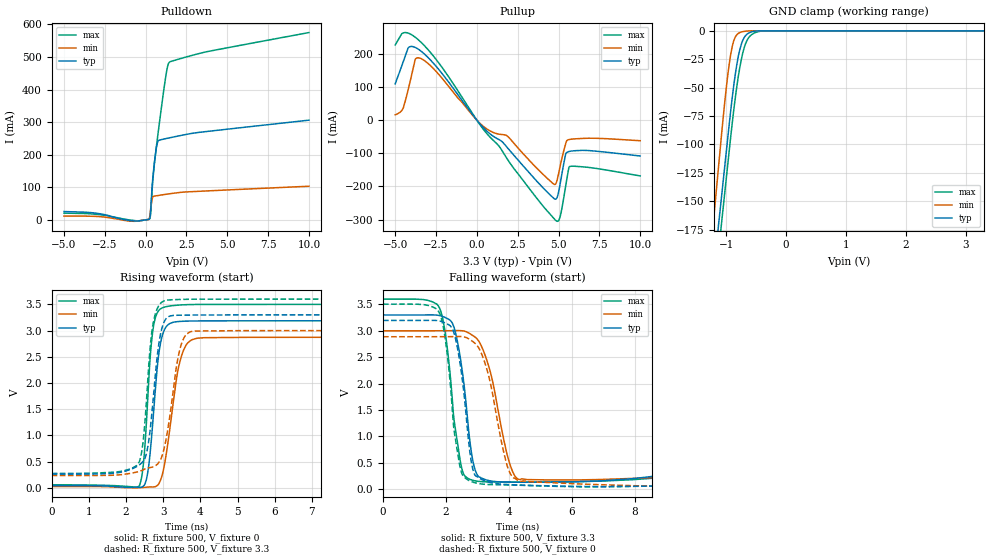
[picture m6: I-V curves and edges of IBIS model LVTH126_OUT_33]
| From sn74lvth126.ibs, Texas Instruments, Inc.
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[Model]   LVTH126_OUT_33
Model_type  3-state
Enable   Active-High
Vref =   0
Rref =   500
Cref =   50p
Vmeas =   1.5
| variable   typ   min   max
C_comp   3.41pF   2.80pF   4.69pF
| C_pullup   4.02pF   0.55pF   5.35pF
| C_pulldown   8.51pF   2.05pF   35.10pF
| C_tri-state   3.41pF   2.80pF   4.69pF
[Temperature Range]   40   -40   100
| Ambient temperature   25   -40   85
[Voltage range]   3.3   3   3.6
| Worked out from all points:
|   slope of the pulldown table from 0 to 0.495 V, typ, clamps not added: 3.18 ohm
|   slope of the pullup table from 0 to 0.495 V, typ, clamps not added: 17.9 ohm
|   GND clamp passes 1 mA (typ) near -0.58 V on its own axis
|   rising waveform, R_fixture 500, V_fixture 0: 20-80 % time 233ps typ, 344ps min, 188ps max; typ from 0.041 V to 3.19 V
|   falling waveform, R_fixture 500, V_fixture 3.3: 20-80 % time 371ps typ, 596ps min, 368ps max; typ from 3.3 V to 0.26 V
|   rising waveform, R_fixture 500, V_fixture 3.3: 20-80 % time 267ps typ, 353ps min, 220ps max; typ from 0.261 V to 3.3 V
|   falling waveform, R_fixture 500, V_fixture 0: 20-80 % time 369ps typ, 599ps min, 369ps max; typ from 3.2 V to 0.041 V
[GND Clamp]
| LVTH126_OUT_33
|   Voltage   I(typ)   I(min)   I(max)
-5.5V     -2.861A    -3.034A    -2.892A
-1.24V    -226.4mA   -182.9mA   -251mA
-1.21V    -211.3mA   -165.7mA   -235.5mA
-1.17V    -191.4mA   -142.9mA   -215.1mA
-1.075V   -144mA     -89.19mA   -167.4mA
-975mV    -94.37mA   -39.09mA   -117.7mA
-925mV    -69.94mA   -20.46mA   -92.96mA
-875mV    -48.14mA   -8.719mA   -69.85mA
-800mV    -22.75mA   -2.299mA   -40.47mA
-725mV    -8.466mA   -746.4uA   -19.69mA
-575mV    -873.9uA   -11.47uA   -3.26mA
3.3V      32.83pA    25.31pA    1.688nA
[Pulldown]
| LVTH126_OUT_33
|   Voltage   I(typ)   I(min)   I(max)
-5V       25.27mA    11.42mA    20.38mA
-3.085V   20.58mA    10.43mA    17.13mA
-705mV    -3.69mA    -4.657mA   -2.29mA
250mV     4.096mA    9.458mA    3.679mA
315mV     33.12mA    35.96mA    22.65mA
425mV     118.9mA    68.08mA    110mA
580mV     192.7mA    73.08mA    190.3mA
710mV     233.6mA    74.13mA    244.7mA
1.24V     249.3mA    78.23mA    442mA
1.36V     250.6mA    79.11mA    473.7mA
1.465V    251.7mA    79.87mA    484.4mA
10V       306mA      103.1mA    575.1mA
[Pullup]
| LVTH126_OUT_33
|   Voltage   I(typ)   I(min)   I(max)
-5V       110.1mA    16.64mA    227.5mA
-4.535V   173.3mA    34.41mA    263.2mA
-4.2V     218.9mA    93.95mA    263.1mA
-3.775V   219.9mA    183.8mA    250.7mA
-3.445V   209.6mA    186.9mA    236.7mA
260mV     -15.41mA   -12.72mA   -18.54mA
1.855V    -82.19mA   -47.41mA   -116.7mA
4.885V    -235.7mA   -185.5mA   -304.7mA
5.11V     -188.9mA   -136.1mA   -288.5mA
5.435V    -102.2mA   -70.96mA   -199.1mA
5.68V     -93.91mA   -57.89mA   -139.8mA
10V       -107.9mA   -61.81mA   -168.2mA
[Ramp]
| LVTH126_OUT_33
| variable   typ   min   max
dV/dt_r   1.91/2.38E-10   1.72/3.55E-10   2.10/1.92E-10
dV/dt_f   1.90/3.89E-10   1.70/6.11E-10   2.08/3.91E-10
R_load = 500
[Rising Waveform]
| LVTH126_OUT_33
R_fixture =   500
C_fixture =   0
L_fixture =   0
V_fixture =   0
V_fixture_min = 0
V_fixture_max = 0
|   Time   V(typ)   V(min)   V(max)
0s        41.24mV    24.56mV    57mV
2.36ns    10.18mV    941.8uV    40.3mV
2.465ns   31.77mV    5.651mV    442.3mV
2.57ns    234.3mV    12.17mV    1.515V
2.755ns   1.564V     17.13mV    3.143V
2.955ns   2.848V     200.1mV    3.426V
3.305ns   3.164V     1.809V     3.48V
3.595ns   3.179V     2.696V     3.493V
4.105ns   3.185V     2.864V     3.499V
50ns      3.188V     2.873V     3.5V
[Falling Waveform]
| LVTH126_OUT_33
R_fixture =   500
C_fixture =   0
L_fixture =   0
V_fixture =   3.3
V_fixture_min = 3
V_fixture_max = 3.6
|   Time   V(typ)   V(min)   V(max)
0s        3.3V       3V         3.6V
1.75ns    3.294V     3.001V     3.478V
1.98ns    3.251V     3.001V     2.95V
2.205ns   3.144V     3.002V     1.676V
2.53ns    2.187V     2.999V     334.1mV
2.81ns    690.5mV    2.927V     175.3mV
3.025ns   245.2mV    2.819V     148.1mV
3.995ns   133.2mV    542.3mV    135.5mV
4.33ns    130.9mV    183.6mV    135.1mV
50ns      260.2mV    234.4mV    273.1mV
[Rising Waveform]
| LVTH126_OUT_33
R_fixture =   500
C_fixture =   0
L_fixture =   0
V_fixture =   3.3
V_fixture_min = 3
V_fixture_max = 3.6
|   Time   V(typ)   V(min)   V(max)
0s        260.8mV    234.8mV    273.5mV
2.325ns   421.5mV    307.4mV    457.7mV
2.445ns   493.2mV    337.1mV    801.8mV
2.555ns   672.1mV    369.5mV    1.718V
2.735ns   1.729V     401.8mV    3.157V
2.92ns    2.903V     526.9mV    3.513V
3.15ns    3.267V     1.236V     3.584V
3.47ns    3.293V     2.698V     3.594V
3.86ns    3.296V     2.991V     3.599V
50ns      3.3V       3V         3.6V
[Falling Waveform]
| LVTH126_OUT_33
R_fixture =   500
C_fixture =   0
L_fixture =   0
V_fixture =   0
V_fixture_min = 0
V_fixture_max = 0
|   Time   V(typ)   V(min)   V(max)
0s        3.196V     2.888V     3.505V
1.745ns   3.192V     2.888V     3.386V
1.97ns    3.15V      2.889V     2.877V
2.19ns    3.053V     2.889V     1.609V
2.5ns     2.164V     2.89V      303.1mV
2.825ns   455.4mV    2.808V     139.9mV
3.145ns   179.5mV    2.546V     96.89mV
3.94ns    88.44mV    451.7mV    79.68mV
4.37ns    76.83mV    149.3mV    73.33mV
50ns      41.25mV    24.55mV    57.08mV
